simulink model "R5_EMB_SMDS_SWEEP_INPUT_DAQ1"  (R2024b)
settings: Solver=ode5  StartTime=0.0  StopTime=S  FixedStep=T  RelTol=1e-3  EnableMultiTasking=on
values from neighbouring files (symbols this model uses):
  Kt = Kt*motor_eff    (= 0.0273)    [R5_EMB_SMDS_SWEEP_INPUT_DAQ1_script.m]
  r = 0.01    [R5_EMB_SMDS_SWEEP_INPUT_DAQ1_script.m]
  S = 30    [R5_EMB_SMDS_SWEEP_INPUT_DAQ1_script.m]
  T = 0.002    [R5_EMB_SMDS_SWEEP_INPUT_DAQ1_script.m]
undefined symbols (not defined in the file or in its folder): Serial_Port, Standard_Devices
libraries: easyio x6, simulink x5

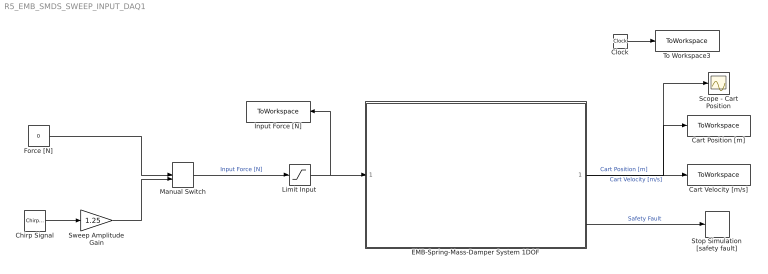
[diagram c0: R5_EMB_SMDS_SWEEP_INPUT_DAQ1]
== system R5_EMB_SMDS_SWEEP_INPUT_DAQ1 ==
  Cart Position [m] : ToWorkspace  VariableName=cart_position  SampleTime=T
  Cart Velocity [m/s] : ToWorkspace  VariableName=cart_velocity  SampleTime=T
  Chirp Signal : simulink/Sources/Chirp Signal  f1=0  T=S  f2=10
  Clock : Clock
  EMB-Spring-Mass-Damper System 1DOF : Subsystem
  Force [N] : Constant  Value=0  SampleTime=T
  Input Force [N] : ToWorkspace  VariableName=f_input  SampleTime=T
  Limit Input : Saturate  UpperLimit=10  LowerLimit=-10
  Manual Switch : ManualSwitch  CurrentSetting=0
  Scope - Cart Position : Scope
  Stop Simulation [safety fault] : Stop
  Sweep Amplitude Gain : Gain  Gain=1.25
  To Workspace3 : ToWorkspace  VariableName=rt_time  SampleTime=T
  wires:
  Clock/1 -> To Workspace3/1
  EMB-Spring-Mass-Damper System 1DOF/1(Out1) -> Scope - Cart Position/1, Cart Position [m]/1  "Cart Position [m]"
  EMB-Spring-Mass-Damper System 1DOF/3(Out3) -> Stop Simulation [safety fault]/1  "Safety Fault"
  EMB-Spring-Mass-Damper System 1DOF/2(Out2) -> Cart Velocity [m/s]/1  "Cart Velocity [m/s]"
  Limit Input/1 -> Input Force [N]/1, EMB-Spring-Mass-Damper System 1DOF/1(In1)
  Manual Switch/1 -> Limit Input/1  "Input Force [N]"
  Force [N]/1 -> Manual Switch/1
  Chirp Signal/1 -> Sweep Amplitude Gain/1
  Sweep Amplitude Gain/1 -> Manual Switch/2

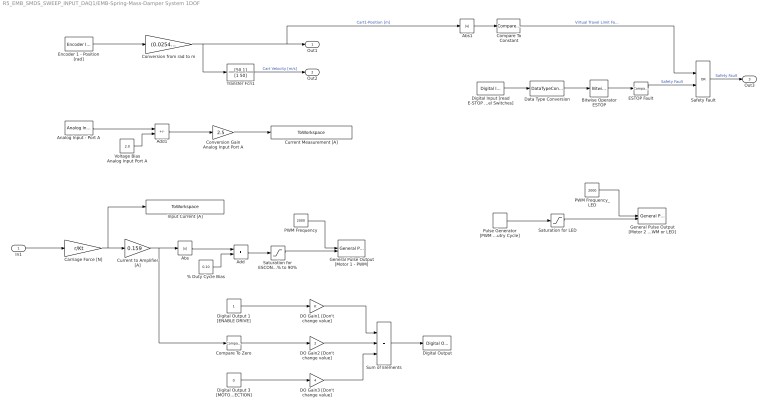
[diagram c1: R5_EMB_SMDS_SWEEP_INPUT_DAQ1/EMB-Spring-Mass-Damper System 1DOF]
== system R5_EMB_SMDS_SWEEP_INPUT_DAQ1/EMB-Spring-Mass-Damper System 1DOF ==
  In1 : Inport
  % Duty Cycle Bias : Constant  Value=0.10  SampleTime=T
  Abs : Abs
  Abs1 : Abs
  Add : Sum
  Add1 : Sum  Inputs=+-
  Analog Input - Port A : easyio/Analog Input  SampleTime=T  MaxMissedTicks=10  ShowMissedTicks=0  YieldWhenWaiting=0  DrvName=Standard_Devices/Serial_Port  DrvAddress=6  DrvOptions=[460800 8 0 0 0 0 0 0]  PacketSize=8  DataTypes='double'  ShowReady=0  ShowError=0  PacketID=1  ByteOrder=1  ShowTimestamp=0  CfgPrm=A6  PrmCfg=unipolar  ResVar=0  VarRes=0
  Bitwise Operator ESTOP : simulink/Logic and Bit Operations/Bitwise Operator  logicop=AND  UseBitMask=on  BitMask=8  BitMaskRealWorld=Real World Value
  Carriage Force [N] : Gain  Gain=r/Kt
  Compare To Constant : simulink/Logic and Bit Operations/Compare To Constant  relop=>=  const=0.035  OutDataTypeStr=boolean
  Compare To Zero : simulink/Logic and Bit Operations/Compare To Zero  relop=>=  OutDataTypeStr=boolean
  Conversion Gain Analog Input Port A : Gain  Gain=2.5
  Conversion from rad to m : Gain  Gain=(0.0254)/(2*pi)
  Current Measurement [A] : ToWorkspace  VariableName=i_measure  SampleTime=T
  Current to Amplifier [A] : Gain  Gain=0.159
  DO Gain1 [Don't change value] : Gain
  DO Gain2 [Don't change value] : Gain  Gain=2
  DO Gain3 [Don't change value] : Gain  Gain=4
  Data Type Conversion : DataTypeConversion  OutDataTypeStr=uint8  RndMeth=Nearest
  Digital Input [read E-STOP and End of Travel Switches] : easyio/Digital Input  SampleTime=T  MaxMissedTicks=10  ShowMissedTicks=0  YieldWhenWaiting=0  DrvName=Standard_Devices/Serial_Port  DrvAddress=6  DrvOptions=[460800 8 0 0 0 0 0 0]  PacketSize=8  DataTypes='double'  ShowReady=0  ShowError=0  PacketID=1  ByteOrder=1  ShowTimestamp=0  CfgPrm=D0  PrmCfg=18  ResVar=0  VarRes=0  d7=off  d6=off  d5=off  d4=on  d3=on  d2=off  d1=off  d0=off
  Digital Output : easyio/Digital Output  SampleTime=T  MaxMissedTicks=10  ShowMissedTicks=0  YieldWhenWaiting=0  DrvName=Standard_Devices/Serial_Port  DrvAddress=6  DrvOptions=[460800 8 0 0 0 0 0 0]  PacketSize=8  DataTypes='double'  ShowReady=0  ShowError=0  PacketID=1  ByteOrder=1  InitialValue=0  FinalValue=0  CfgPrm=G0  PrmCfg=F8  ResVar=0  VarRes=0  d7=off  d6=off  d5=off  d4=off  d3=off  d2=on  d1=on  d0=on
  Digital Output 1 [ENABLE DRIVE] : Constant  SampleTime=T
  Digital Output 3 [MOTOR 2 DIRECTION] : Constant  Value=0  SampleTime=T
  ESTOP Fault : simulink/Logic and Bit Operations/Compare To Constant  relop=~=  const=8  OutDataTypeStr=boolean
  Encoder 1 - Position [rad] : easyio/Encoder Input  SampleTime=T  MaxMissedTicks=10  ShowMissedTicks=0  YieldWhenWaiting=0  DrvName=Standard_Devices/Serial_Port  DrvAddress=6  DrvOptions=[460800 8 0 0 0 0 0 0]  PacketSize=8  DataTypes='double'  ShowReady=0  ShowError=0  PacketID=1  ByteOrder=1  ShowTimestamp=0  CfgPrm=E0  PrmCfg=position  ResVar=0  VarRes=2000
  General Pulse Output [Motor 1 - PWM] : easyio/General Pulse Output  SampleTime=T  MaxMissedTicks=10  ShowMissedTicks=0  YieldWhenWaiting=0  DrvName=Standard_Devices/Serial_Port  DrvAddress=6  DrvOptions=[460800 8 0 0 0 0 0 0]  PacketSize=16  DataTypes={'double','double'}  ShowReady=0  ShowError=0  PacketID=1  ByteOrder=1  InitialValue=[0 0]  FinalValue=[0 0]  CfgPrm=N0  PrmCfg=frequency and duty  ResVar=449.8360 Hz - 115156.25 Hz  VarRes=64
  General Pulse Output [Motor 2 - PWM or LED] : easyio/General Pulse Output  SampleTime=T  MaxMissedTicks=10  ShowMissedTicks=0  YieldWhenWaiting=0  DrvName=Standard_Devices/Serial_Port  DrvAddress=6  DrvOptions=[460800 8 0 0 0 0 0 0]  PacketSize=16  DataTypes={'double','double'}  ShowReady=0  ShowError=0  PacketID=1  ByteOrder=1  InitialValue=[0 0]  FinalValue=[0 0]  CfgPrm=N1  PrmCfg=frequency and duty  ResVar=449.8360 Hz - 115156.25 Hz  VarRes=64
  Input Current [A] : ToWorkspace  VariableName=i_input  SampleTime=T
  PWM Frequency : Constant  Value=2000  SampleTime=T
  PWM Frequency_LED : Constant  Value=2000  SampleTime=T
  Pulse Generator [PWM % Dutry Cycle] : DiscretePulseGenerator  PulseType=Time based  Period=0.4  PulseWidth=50
  Safety Fault : Logic  Operator=OR  AllPortsSameDT=off  OutDataTypeStr=boolean
  Saturation for ESCON 10% to 90% : Saturate  UpperLimit=0.9  LowerLimit=0.1
  Saturation for LED : Saturate  UpperLimit=1  LowerLimit=0
  Sum of Elements : Sum  Inputs=+++
  Transfer Fcn1 : TransferFcn  Numerator=[50 1]  Denominator=[1 50]
  Voltage Bias Analog Input Port A : Constant  Value=2.0
  Out1 : Outport
  Out2 : Outport  Port=2
  Out3 : Outport  Port=3
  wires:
  % Duty Cycle Bias/1 -> Add/2
  Conversion Gain Analog Input Port A/1 -> Current Measurement [A]/1
  Add1/1 -> Conversion Gain Analog Input Port A/1
  Current to Amplifier [A]/1 -> Abs/1, Compare To Zero/1
  Saturation for ESCON 10% to 90%/1 -> General Pulse Output [Motor 1 - PWM]/2
  Voltage Bias Analog Input Port A/1 -> Add1/2
  DO Gain2 [Don't change value]/1 -> Sum of Elements/2
  Analog Input - Port A/1 -> Add1/1
  PWM Frequency/1 -> General Pulse Output [Motor 1 - PWM]/1
  DO Gain1 [Don't change value]/1 -> Sum of Elements/1
  Digital Output 1 [ENABLE DRIVE]/1 -> DO Gain1 [Don't change value]/1
  Saturation for LED/1 -> General Pulse Output [Motor 2 - PWM or LED]/2
  PWM Frequency_LED/1 -> General Pulse Output [Motor 2 - PWM or LED]/1
  Carriage Force [N]/1 -> Input Current [A]/1, Current to Amplifier [A]/1
  Pulse Generator [PWM % Dutry Cycle]/1 -> Saturation for LED/1
  Encoder 1 - Position [rad]/1 -> Conversion from rad to m/1
  Sum of Elements/1 -> Digital Output/1
  Add/1 -> Saturation for ESCON 10% to 90%/1
  Compare To Zero/1 -> DO Gain2 [Don't change value]/1
  Abs/1 -> Add/1
  In1/1 -> Carriage Force [N]/1
  Digital Output 3 [MOTOR 2 DIRECTION]/1 -> DO Gain3 [Don't change value]/1
  DO Gain3 [Don't change value]/1 -> Sum of Elements/3
  Transfer Fcn1/1 -> Out2/1  "Cart Velocity [m/s]"
  Bitwise Operator ESTOP/1 -> ESTOP Fault/1
  Data Type Conversion/1 -> Bitwise Operator ESTOP/1
  Digital Input [read E-STOP and End of Travel Switches]/1 -> Data Type Conversion/1
  Abs1/1 -> Compare To Constant/1
  Compare To Constant/1 -> Safety Fault/1  "Virtual Travel Limit Fault"
  Conversion from rad to m/1 -> Abs1/1, Out1/1, Transfer Fcn1/1  "Cart1-Position [m]"
  Safety Fault/1 -> Out3/1  "Safety Fault"
  ESTOP Fault/1 -> Safety Fault/2  "Safety Fault"
